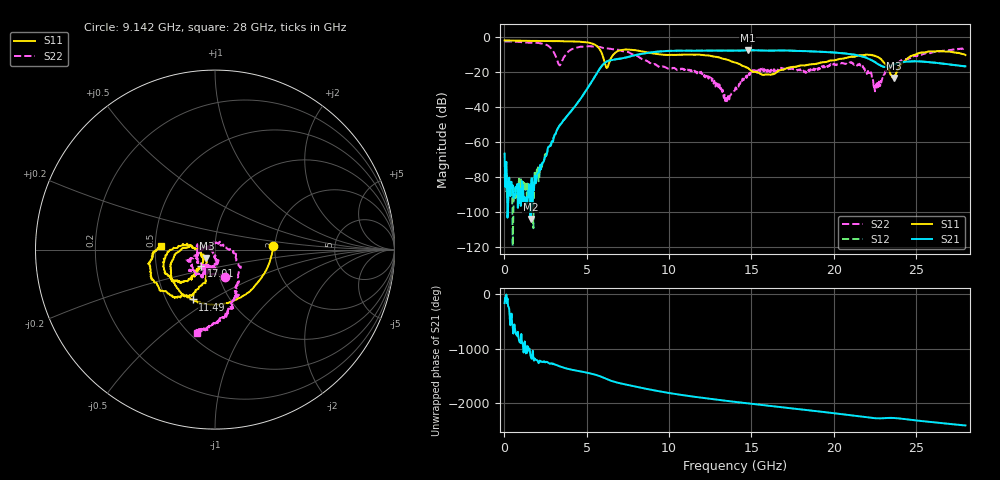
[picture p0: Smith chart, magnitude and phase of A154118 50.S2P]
!  2-Port S-parameters saved by WinCal
! VAR MeasName=S-Parameters (CALIBRATED_DATA) read from VNA (N5230A)
! VAR MeasDate=2015-9-10 14:38:29
! VAR NAME=A154118 50
! VAR FILENAME=A154118 50.S2P
! VAR DATE=2015-9-10 14:38:29
! VAR PHYS_PORTS=1,2
# Hz S DB R 50
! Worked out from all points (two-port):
!   801 points, 10 MHz to 28 GHz, reference 50 ohm
!   highest |S21| = -7.74 dB at 14.77 GHz (marker M1); lowest = -104.1 dB at 1.584 GHz (marker M2)
!   |S21| within 3 dB of the highest: 7.844 GHz to 21.48 GHz (13.64 GHz wide, 93 % of centre)
!   lowest |S11| = -23.5 dB at 23.66 GHz (marker M3), VSWR 1.14, Z = 45.2 - j4.18 ohm
!   |S11| at or under -10 dB: 5.934 GHz to 6.639 GHz (704.8 MHz wide, 11.2 % of centre); 9.314 GHz to 25.02 GHz (15.71 GHz wide, 91.5 % of centre); 27.89389 GHz to end of sweep
!   |S22| runs from -36.8 to -2.7 dB; largest |S21 - S12| = 0.0081
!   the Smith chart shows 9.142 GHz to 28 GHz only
!   S11 on the Smith chart (normalised r, x): 9.142 GHz: 1.96, +0.08; 11.49 GHz: 0.68, -0.41; 17.01 GHz: 0.85, -0.15; 28 GHz: 0.54, +0.02
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1e7  -2.16 179.7  -66.83 -166.4  -78.37 -3.2  -2.67 179.8
2.899e8  -2.19 175.7  -80.51 91.6  -84.03 107.1  -2.71 172.9
1.584438e9  -2.41 159.2  -104.13 -45.2  -85.93 -23.7  -3.44 142.0
3.053912e9  -2.52 137.3  -55.91 153.8  -56.07 153.9  -9.84 38.5
3.578725e9  -2.63 127.5  -47.68 95.7  -47.83 95.6  -12.31 -124.8
4.698325e9  -3.01 98.3  -34.43 22.2  -34.42 22.1  -5.69 147.7
5.677975e9  -5.88 36.1  -19.85 -49.1  -19.79 -49.2  -5.85 108.2
6.132812e9  -16.19 -59.8  -14.64 -104.8  -14.56 -104.9  -6.66 92.7
7.357375e9  -7.30 94.3  -11.94 145.8  -11.94 145.6  -8.52 40.3
9.141738e9  -9.76 3.3  -8.70 37.0  -8.68 36.7  -15.89 -69.2
9.351662e9  -10.03 -8.6  -8.53 25.4  -8.48 25.3  -17.12 -80.5
1.14859e10  -10.33 -114.1  -8.00 -76.0  -7.95 -76.4  -20.04 -162.7
1.4005e10  -14.72 177.9  -7.94 -170.6  -7.92 -171.2  -30.46 -96.4
1.477472e10  -17.87 172.4  -7.74 162.5  -7.69 161.9  -21.54 -81.3
1.701392e10  -18.62 -130.4  -7.92 85.9  -7.89 85.4  -18.22 -119.9
1.869332e10  -15.66 -128.9  -8.38 28.2  -8.39 27.8  -18.13 -108.7
2.159729e10  -10.65 -144.2  -11.00 -76.9  -10.88 -78.0  -15.85 -155.3
2.257694e10  -11.11 -173.4  -14.96 -110.1  -14.92 -111.2  -27.07 100.8
2.334666e10  -19.09 176.7  -17.09 -103.6  -17.05 -104.8  -17.92 -13.3
2.366155e10  -23.50 -136.4  -15.89 -105.5  -15.86 -106.3  -15.31 -33.3
2.5201e10  -9.42 -128.7  -14.09 -155.9  -14.10 -157.4  -10.45 -68.9
2.8e10  -10.47 176.4  -16.90 118.6  -17.02 117.6  -6.47 -102.3
